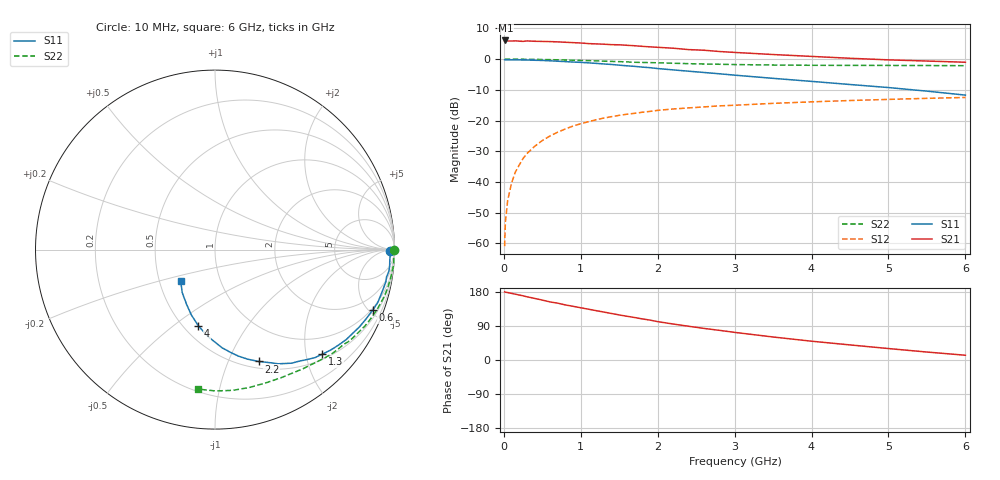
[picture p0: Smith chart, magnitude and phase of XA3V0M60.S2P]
! SIEMENS Discrete & RF Semiconductors
! BFY180
! Si NPN RF Bipolar Junction Transistor in MICRO-X
! VCE = 3 V  IC = 0.6 mA
! Common Emitter S-Parameters:  May  1997
# GHz  S  MA  R  50
!  f  S11  S21  S12  S22
! GHz  MAG  ANG  MAG  ANG  MAG  ANG  MAG  ANG
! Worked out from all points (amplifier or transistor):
!   36 points, 10 MHz to 6 GHz, reference 50 ohm
!   highest |S21| = 6.1 dB at 20 MHz (marker M1)
!   |S21| within 3 dB of that: start of sweep to 2.424 GHz
!   unconditionally stable (mu >= 1): 4.895 GHz to end of sweep
!   at 250 MHz: K = 0.05, MSG = 19.1 dB, |S12| = -32.4 dB
!   at 1.4 GHz: K = 0.42, MSG = 11.7 dB, |S12| = -18.7 dB
!   at 6 GHz: K = 1.03, MAG = 4.7 dB, |S12| = -12.5 dB
!   S11 on the Smith chart (normalised r, x): 10 MHz: 80, -18; 600 MHz: 0.89, -5.22; 1.3 GHz: 0.60, -2.33; 2.2 GHz: 0.57, -1.30; 4 GHz: 0.59, -0.62; 6 GHz: 0.64, -0.24
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0.01  0.9765 -0.3  1.965 179.7  0.0009 84.0  0.9984 -0.1
0.02  0.9755 -0.6  2.017 179.0  0.0022 90.9  0.9999 -0.5
0.05  0.9764 -1.7  1.978 178.0  0.005 85.1  0.9979 -1.2
0.1  0.9758 -3.6  1.975 175.8  0.0096 87.2  0.9955 -2.4
0.15  0.9773 -5.4  1.986 173.7  0.0145 86.8  0.9978 -3.6
0.25  0.9676 -9.1  1.949 169.4  0.0241 84.2  0.9969 -6.0
0.3  0.9689 -10.6  1.981 166.8  0.029 82.1  0.9937 -7.0
0.6  0.9407 -21.1  1.933 153.3  0.0561 74.3  0.9819 -14.0
0.8  0.913 -28.1  1.885 145.3  0.073 68.9  0.968 -18.5
1.1  0.8704 -37.6  1.793 134.1  0.0958 61.2  0.9457 -24.9
1.3  0.8353 -44.2  1.753 126.5  0.1099 56.8  0.9278 -28.9
1.5  0.7987 -50.1  1.713 118.9  0.1217 52.4  0.9113 -32.8
1.7  0.7634 -56.0  1.654 112.1  0.1312 48.8  0.8903 -36.4
2  0.7035 -63.7  1.559 101.2  0.1467 43.6  0.8729 -41.5
2.2  0.6689 -68.7  1.509 95.0  0.1542 40.2  0.8586 -44.8
2.6  0.607 -77.7  1.398 83.4  0.1668 34.9  0.8334 -50.6
3  0.5491 -85.8  1.288 72.9  0.1775 29.9  0.8167 -56.2
3.5  0.4871 -94.4  1.19 60.7  0.1907 24.8  0.8032 -62.7
4  0.4348 -102.3  1.109 49.6  0.2017 19.9  0.7947 -69.3
4.5  0.3866 -110.0  1.034 39.8  0.2121 15.5  0.7917 -76.0
5.5  0.3014 -127.3  0.932 21.0  0.23 6.9  0.7877 -89.8
6  0.2599 -137.3  0.891 12.6  0.2379 2.3  0.7828 -96.8
